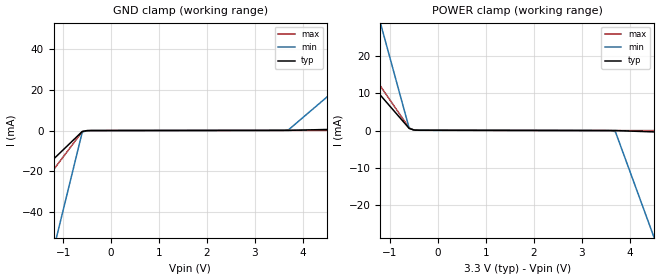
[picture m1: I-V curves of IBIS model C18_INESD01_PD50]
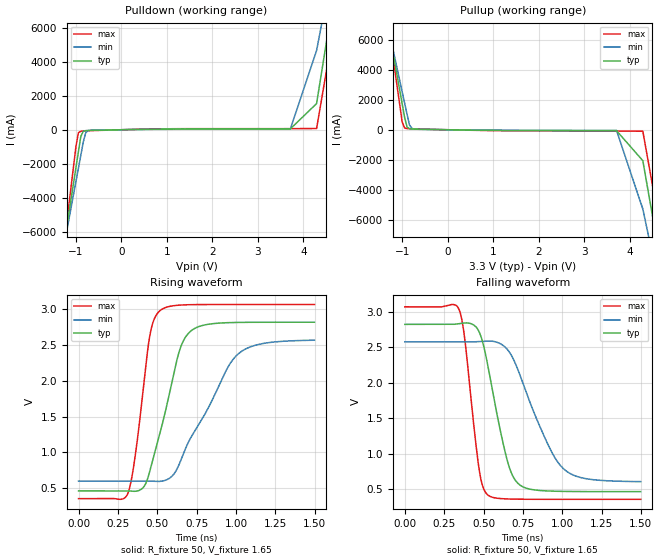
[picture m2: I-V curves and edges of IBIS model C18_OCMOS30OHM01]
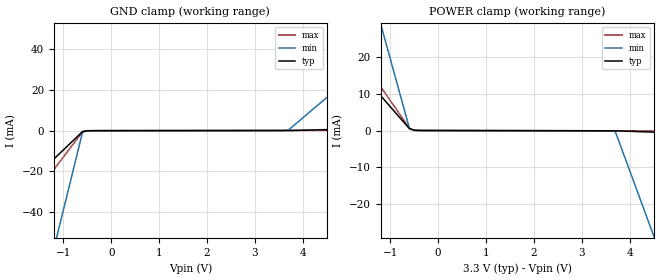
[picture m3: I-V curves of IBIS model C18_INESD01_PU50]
|   This file is an IBIS representation of the   |
|   Integrated Device Technology, Inc.   |
|   ICS813N2532I   |
|   JITTER ATTENUATOR/MULTIPLIER & FEMTOCLOCK NG MULTIPLIER   |
[IBIS Ver]   4.1
[File name]   813n2532i_3v3.ibs
[File Rev]   1.0
[Date]   20 Aug 2010
[Source]   Originated at Integrated Device Technology, Inc.
[Disclaimer]
IDT hereby grants the user of this IBIS model a non-exclusive,
nontransferable license to use this IBIS model under the following terms.
Before using this IBIS model, the user should read this license.
If the user does not accept these terms,  the IBIS model should be
returned to IDT within 30 days.
   The user is granted this license only to use the IBIS model and
is not granted rights to sell, load, rent, lease or license the IBIS
model in whole or in part, or in modified form to anyone other than
user. User may modify the IBIS model to suit its specific
applications but rights to derivative works and such modifications
shall belong to IDT.
   This IBIS model is provided on an "AS IS" basis and IDT makes
absolutely no warranty with respect to the information contained
herein. IDT DISCLAIMS AND CUSTOMER WAIVES ALL WARRANTIES, EXPRESS
OR IMPLIED, INCLUDING WARRANTIES OF MERCHANTABILITY OR FITNESS FOR
A PARTICULAR PURPOSE. The entire risk as to quality and performance
is with the Customer. ACCORDINGLY, IN NO EVENT SHALL THE COMPANY BE
LIABLE FOR ANY DAMAGES, WHETHER IN CONTRACT OR TORT,INCLUDING ANY
LOST PROFITS OR OTHER INCIDENTAL, CONSEQUENTIAL, EXEMPLARY, OR
PUNITIVE DAMAGES ARISING OUT OF THE USE OR APPLICATION OF THE IBIS
model provided in this package. Further, IDT reserves the right to
make changes without notice to any product herein to improve
reliability, function, or design. IDT does not convey any license
under patent rights or any other intellectual property rights,
including those of third parties.
   IDT is not obligated to provide maintenance or support
for the licensed IBIS model.
[Copyright]   Copyright 2010 by Integrated Device Technology, Inc.
[Component]   ICS813N2532KI
[Manufacturer] Integrated Device Technology, Inc.
[Package]
|QFN 32
|lead + wire   typ   min   max
R_pkg   72.4655m   58.886m   86.045m
L_pkg   1.47175nH   1.11650nH   1.77850nH
C_pkg   0.07747pF   0.07444pF   0.08050pF
[Pin] signal_name   model_name   R_pin   L_pin   C_pin
1   LF1   NC   86.045m   1.77850nH   0.08050pF
2   LF0   NC   76.996m   1.55783nH   0.07848pF
3   ISET   NC   67.941m   1.33717nH   0.07646pF
4   VEE   GND   58.886m   1.11650nH   0.07444pF
5   CLK_SEL   C18_INESD01_PD50   58.886m   1.11650nH   0.07444pF
6   VCC   POWER   67.941m   1.33717nH   0.07646pF
7   LOR   C18_OCMOS30OHM01   76.996m   1.55783nH   0.07848pF
8   VEE   GND   86.045m   1.77850nH   0.08050pF
9   FB_SEL   C18_INESD01_PU50   86.045m   1.77850nH   0.08050pF
10   PDSEL_1   C18_INESD01_PU50   76.996m   1.55783nH   0.07848pF
11   PDSEL_0   C18_INESD01_PU50   67.941m   1.33717nH   0.07646pF
12   VCC   POWER   58.886m   1.11650nH   0.07444pF
13   VCCA   POWER   58.886m   1.11650nH   0.07444pF
14   ODBSEL_1   C18_INESD01_PD50   67.941m   1.33717nH   0.07646pF
15   ODBSEL_0   C18_INESD01_PD50   76.996m   1.55783nH   0.07848pF
16   ODASEL_1   C18_INESD01_PD50   86.045m   1.77850nH   0.08050pF
17   ODASEL_0   C18_INESD01_PD50   86.045m   1.77850nH   0.08050pF
18   VEE   GND   76.996m   1.55783nH   0.07848pF
19   QA   C18_OHSUNIV01_OE   67.941m   1.33717nH   0.07646pF
20   nQA   C18_OHSUNIV01_OE   58.886m   1.11650nH   0.07444pF
21   VCCO   POWER   58.886m   1.11650nH   0.07444pF
22   QB   C18_OHSUNIV01_OE   67.941m   1.33717nH   0.07646pF
23   nQB   C18_OHSUNIV01_OE   76.996m   1.55783nH   0.07848pF
24   VEE   GND   86.045m   1.77850nH   0.08050pF
25   nCLK1   C18_nINDIFF01PDP   86.045m   1.77850nH   0.08050pF
26   CLK1   C18_INDIFF01PDPU   76.996m   1.55783nH   0.07848pF
27   VCC   POWER   67.941m   1.33717nH   0.07646pF
28   nCLK0   C18_nINDIFF01PDP   58.886m   1.11650nH   0.07444pF
29   CLK0   C18_INDIFF01PDPU   58.886m   1.11650nH   0.07444pF
30   XTAL_OUT   NC   67.941m   1.33717nH   0.07646pF
31   XTAL_IN   NC   76.996m   1.55783nH   0.07848pF
32   VCCX   POWER   86.045m   1.77850nH   0.08050pF
[Diff Pin]  inv_pin  vdiff tdelay_typ tdelay_min  tdelay_max
|Input
26   25   0.15  0   0   0
29   28   0.15  0   0   0
|Output
19   20   NA   0   0   0
22   23   NA   0   0   0
| Models and submodels in the file (6): C18_INESD01_PD50 (Input), C18_OCMOS30OHM01 (Output), C18_INESD01_PU50 (Input), C18_OHSUNIV01_OE (Output_ECL), C18_nINDIFF01PDP (Input), C18_INDIFF01PDPU (Input)
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[Model]   C18_INESD01_PD50
Model_type   Input
Polarity   Non-Inverting
Vinl = 0.8V
Vinh = 2.2V
|   typ   min   max
C_comp   2pF   1.5pF   2.5pF
|   typ   min   max
[Voltage range]   3.3V   3.135V   3.465V
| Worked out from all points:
|   GND clamp passes 1 mA (typ) near -0.62 V on its own axis
|   POWER clamp passes 1 mA (typ) near -0.63 V on its own axis
[GND_clamp]
|Voltage   I (typ)   I (min)   I (max)
-3.3V     -61.32mA   -259.6mA   -84.4mA
-2.9V     -52.31mA   -221.3mA   -71.97mA
-2.8V     -50.05mA   -211.7mA   -68.87mA
-2.3V     -38.78mA   -163.7mA   -53.33mA
-2.2V     -36.52mA   -154.1mA   -50.23mA
-1.2V     -13.98mA   -58.24mA   -19.17mA
-1.1V     -11.73mA   -48.65mA   -16.06mA
-600mV    -453.3uA   -698.6uA   -527.7uA
-400mV    -11.1uA    -13uA      -9.761uA
3.7V      77.31uA    339.6uA    78.55uA
6.2V      1.427mA    50.43mA    134.4uA
6.6V      1.643mA    58.44mA    143.4uA
[Power_clamp]
|Voltage   I (typ)   I (min)   I (max)
-3.3V     40.74mA    127.9mA    51.33mA
-2.5V     28.83mA    90.18mA    36.32mA
-2.4V     27.35mA    85.47mA    34.44mA
-2.1V     22.88mA    71.33mA    28.82mA
-2V       21.4mA     66.62mA    26.94mA
-1.2V     9.494mA    28.91mA    11.94mA
-1.1V     8.006mA    24.2mA     10.06mA
-600mV    567.9uA    633.8uA    683uA
-500mV    131.3uA    131.4uA    134.2uA
3.7V      -11.1uA    -299.6uA   -4.991uA
4.5V      -367.9uA   -28.5mA    -22.78uA
6.6V      -1.304mA   -102.5mA   -69.48uA
[Model]   C18_OCMOS30OHM01
Model_type   Output
Polarity   Non-Inverting
|   typ   min   max
C_comp   2pF   1.5pF   2.5pF
Vmeas = 1.72V
Rref = 50
Cref = 0
Vref = 1.65V
|   typ   min   max
[Voltage range]   3.3V   3.135V   3.465V
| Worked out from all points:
|   slope of the pulldown table from 0 to 0.495 V, typ, clamps not added: 19.8 ohm
|   slope of the pullup table from 0 to 0.495 V, typ, clamps not added: 20.5 ohm
|   rising waveform, R_fixture 50, V_fixture 1.65: 20-80 % time 156ps typ, 276ps min, 88.6ps max; typ from 0.463 V to 2.82 V
|   falling waveform, R_fixture 50, V_fixture 1.65: 20-80 % time 129ps typ, 220ps min, 78.9ps max; typ from 2.82 V to 0.463 V
[Pulldown]
|Voltage   I (typ)   I (min)   I (max)
-3.3V     -42.11A    -36.24A    -51.97A
-1.46V    -10.24A    -9.707A    -11.23A
-1V       -2.257A    -3.069A    -1.019A
-945mV    -1.303A    -2.276A    -175.8mA
-891mV    -386.5mA   -1.497A    -87.01mA
-837mV    -93.38mA   -719.3mA   -72.75mA
-783mV    -51.96mA   -167mA     -64.37mA
-674.9mV  -37.97mA   -31.04mA   -51.65mA
3.71V     46.28mA    31.92mA    64.2mA
4.288V    1.542A     4.671A     72.2mA
4.866V    11.24A     12.75A     9.141A
6.6V      40.44A     37.09A     46.46A
[Pullup]
|Voltage   I (typ)   I (min)   I (max)
-3.3V     40.5A      34.81A     50.05A
-1.46V    9.486A     8.986A     10.43A
-999mV    1.734A     2.532A     517.7mA
-945mV    825.7mA    1.777A     110.7mA
-891mV    176.9mA    1.021A     74.95mA
-837mV    68mA       312.8mA    67.34mA
-783mV    50.02mA    88.11mA    61.99mA
-728.9mV  44.22mA    43.76mA    56.96mA
3.71V     -62.13mA   -45.72mA   -85.09mA
4.288V    -2.066A    -5.286A    -100.6mA
4.866V    -12.09A    -13.62A    -9.936A
6.6V      -42.14A    -38.62A    -48.37A
[Ramp]
|   typ   min   max
dV/dt_r   1.891/0.224n   1.58/0.38n   2.179/0.134n
dV/dt_f   1.903/0.191n   1.586/0.324n   2.197/0.116n
R_load =   50.0000
[Rising Waveform]
R_fixture = 50
V_fixture = 1.65   |Vcc_typ
V_fixture_min = 1.5675 |Vcc_min
V_fixture_max = 1.7325 |Vcc_max
C_fixture = 0.0p
| Time   typ   min   max
0s        463.1mV    600.7mV    354.4mV
312.3ps   463.4mV    600.9mV    424mV
361.9ps   458mV      601.1mV    984.9mV
415.9ps   524.5mV    601mV      1.986V
452ps     734.5mV    599.7mV    2.625V
518ps     1.277V     596.3mV    2.985V
639.6ps   2.413V     837.1mV    3.06V
720.7ps   2.711V     1.237V     3.067V
1.024ns   2.819V     2.396V     3.069V
1.498ns   2.822V     2.57V      3.069V
[Falling Waveform]
R_fixture = 50
V_fixture = 1.65   |Vcc_typ
V_fixture_min = 1.5675 |Vcc_min
V_fixture_max = 1.7325 |Vcc_max
C_fixture = 0.0p
| Time   typ   min   max
0s        2.822V     2.574V     3.069V
343.8ps   2.831V     2.574V     3.034V
379.9ps   2.841V     2.574V     2.633V
473ps     2.712V     2.58V      765.3mV
527ps     2.245V     2.587V     416.8mV
648.6ps   920.5mV    2.475V     359.9mV
726.7ps   564.2mV    2.136V     356mV
902.4ps   472.8mV    1.161V     354.5mV
1.012ns   466.1mV    778.3mV    354.4mV
1.498ns   463.2mV    603.9mV    354.4mV
[Model]   C18_INESD01_PU50
Model_type   Input
Polarity   Non-Inverting
Vinl = 0.8V
Vinh = 2.2V
|   typ   min   max
C_comp   2pF   1.5pF   2.5pF
|   typ   min   max
[Voltage range]   3.3V   3.135V   3.465V
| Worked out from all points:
|   GND clamp passes 1 mA (typ) near -0.62 V on its own axis
|   POWER clamp passes 1 mA (typ) near -0.63 V on its own axis
[GND_clamp]
|Voltage   I (typ)   I (min)   I (max)
-3.3V     -61.39mA   -259.7mA   -84.47mA
-2.9V     -52.37mA   -221.3mA   -72.05mA
-2.8V     -50.12mA   -211.7mA   -68.94mA
-2.3V     -38.84mA   -163.8mA   -53.41mA
-2.2V     -36.59mA   -154.2mA   -50.3mA
-1.2V     -14.05mA   -58.3mA    -19.24mA
-1.1V     -11.79mA   -48.71mA   -16.13mA
-600mV    -519.3uA   -757.2uA   -601.3uA
-400mV    -77.06uA   -71.62uA   -83.32uA
3.7V      11.34uA    280.9uA    4.99uA
6.2V      1.361mA    50.37mA    60.87uA
6.6V      1.577mA    58.38mA    69.81uA
[Power_clamp]
|Voltage   I (typ)   I (min)   I (max)
-3.3V     40.67mA    127.8mA    51.25mA
-2.5V     28.77mA    90.12mA    36.25mA
-2.4V     27.28mA    85.41mA    34.37mA
-2.1V     22.82mA    71.27mA    28.74mA
-2V       21.33mA    66.56mA    26.87mA
-1.2V     9.428mA    28.85mA    11.86mA
-1.1V     7.94mA     24.14mA    9.988mA
-600mV    501.9uA    575.2uA    609.4uA
-500mV    65.34uA    72.75uA    60.6uA
3.7V      -77.06uA   -358.2uA   -78.55uA
4.5V      -433.9uA   -28.56mA   -96.35uA
6.6V      -1.37mA    -102.6mA   -143uA
